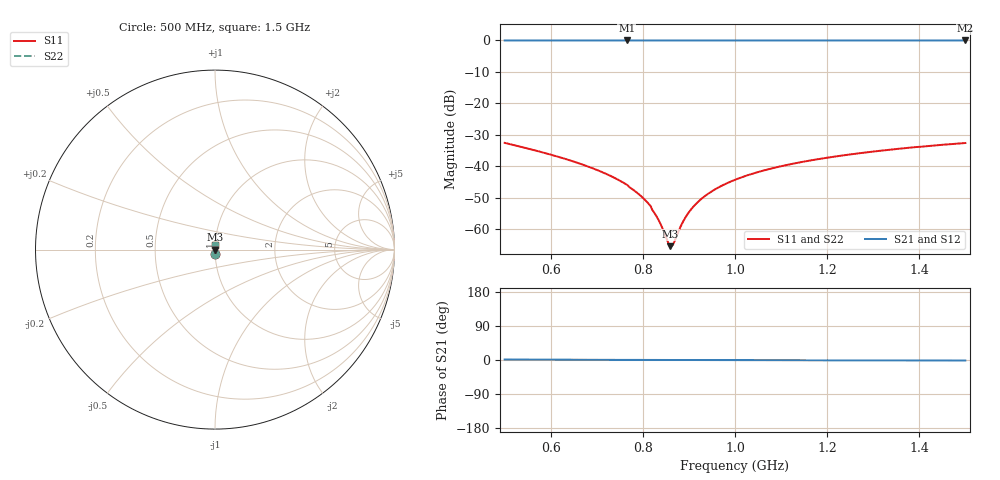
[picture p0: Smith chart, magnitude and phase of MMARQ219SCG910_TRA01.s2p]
! MMARQ219SCG910_TRA01  S-PARAMETER MODEL  ( General Type )
! Model Generated by TAIYO YUDEN Corporation (http://www.ty-top.com)
! Version 1.0
! TAIYO YUDEN Control No. 180601
! Copyright(c) 2018 TAIYO YUDEN CO.,LTD. All Rights Reserved.
! Product Description (link to TY-COMPAS)
! https://ds.yuden.co.jp/TYCOMPAS/or/detail?pn=MMARQ219SCG910JTRA01&u=M
! Products Name : Multilayer Ceramic Capacitors
! Characteristics :
!  Capacitance : 91 pF , Rated Voltage : 250V , TCC : CG / C0G
!  Case Size : 2.0 x 1.25 / 0.079 x 0.049 [mm/inch] , Thickness : 0.85 / 0.033 [mm/inch]
!  (Conditions: Temperature = 25 degC , DC Bias Current/Voltage = 0A / 0V)
! External Node Assignments :
!  1  o---| |---o  2
! GND o---------o GND
! Frequency Range : 500MHz  -  1500MHz  [ 401 STEP ]
# MHz S RI R 50
! Freq[MHz].  S11 Real  S11 Imag  S21 Real  S21 Imag  S12 Real  S12 Imag  S22 Real  S22 Imag
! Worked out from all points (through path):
!   401 points, 500 MHz to 1.5 GHz, reference 50 ohm
!   highest |S21| = 0.00 dB at 765 MHz (marker M1); lowest = 0.0 dB at 1.5 GHz (marker M2)
!   lowest |S11| = -65.4 dB at 860 MHz (marker M3), VSWR 1.00, Z = 50.1 - j0.006 ohm
!   |S11| at or under -10 dB: start of sweep to end of sweep
!   |S22| runs from -65.4 to -32.6 dB; largest |S21 - S12| = 0
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500  0.001 -0.0236  0.999 0.0236  0.999 0.0236  0.001 -0.0236
592.5  0.000716 -0.0159  0.9993 0.0159  0.9993 0.0159  0.000716 -0.0159
667.5  0.000597 -0.0107  0.9994 0.0107  0.9994 0.0107  0.000597 -0.0107
722.5  0.000551 -0.00744  0.9994 0.00744  0.9994 0.00744  0.000551 -0.00744
765  0.000532 -0.00508  0.9995 0.00508  0.9995 0.00508  0.000532 -0.00508
792.5  0.000527 -0.0035  0.9995 0.0035  0.9995 0.0035  0.000527 -0.0035
810  0.000526 -0.00261  0.9995 0.00261  0.9995 0.00261  0.000526 -0.00261
820  0.000527 -0.00199  0.9995 0.00199  0.9995 0.00199  0.000527 -0.00199
835  0.000529 -0.00126  0.9995 0.00126  0.9995 0.00126  0.000529 -0.00126
855  0.000533 -0.000296  0.9995 0.000296  0.9995 0.000296  0.000533 -0.000296
860  0.000535 -6e-05  0.9995 6e-05  0.9995 6e-05  0.000535 -6e-05
862.5  0.000536 5.76e-05  0.9995 -5.76e-05  0.9995 -5.76e-05  0.000536 5.76e-05
867.5  0.000537 0.000292  0.9995 -0.000292  0.9995 -0.000292  0.000537 0.000292
882.5  0.000543 0.000986  0.9995 -0.000986  0.9995 -0.000986  0.000543 0.000986
892.5  0.000547 0.00144  0.9995 -0.00144  0.9995 -0.00144  0.000547 0.00144
915  0.000558 0.00245  0.9994 -0.00245  0.9994 -0.00245  0.000558 0.00245
950  0.000578 0.00398  0.9994 -0.00398  0.9994 -0.00398  0.000578 0.00398
1000  0.000616 0.00607  0.9994 -0.00607  0.9994 -0.00607  0.000616 0.00607
1072.5  0.000684 0.00895  0.9993 -0.00895  0.9993 -0.00895  0.000684 0.00895
1167.5  0.000794 0.0125  0.9992 -0.0125  0.9992 -0.0125  0.000794 0.0125
1335  0.00104 0.0183  0.999 -0.0183  0.999 -0.0183  0.00104 0.0183
1500  0.00132 0.0234  0.9987 -0.0234  0.9987 -0.0234  0.00132 0.0234
